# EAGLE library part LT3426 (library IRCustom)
LT3426 1.2MHz, 2A boost converter in SOT-23 http://www.linear.com/pc/productDetail.jsp?navId=H0,C1,C1003,C1042,C1031,C1061,P8430 (Linear website)
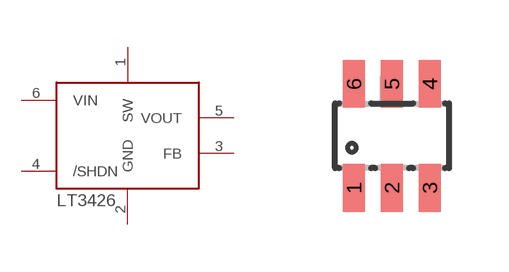
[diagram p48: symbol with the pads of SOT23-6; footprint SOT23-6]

Designator prefix -

## LT3426  [SOT23-6]
1  SW  out
2  GND  sup
3  FB  in
4  /SHDN  in
5  VOUT  out
6  VIN  in

## Footprint SOT23-6 (pad centres in mm)
smd 0.55 x 1.2: 1 -0.95,-1.3; 2 0,-1.3; 3 0.95,-1.3; 4 0.95,1.3; 5 0,1.3; 6 -0.95,1.3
